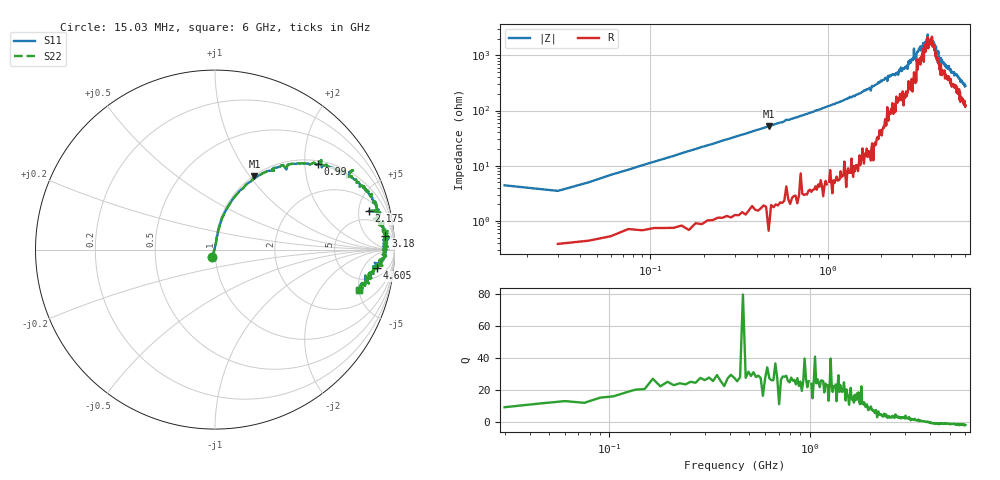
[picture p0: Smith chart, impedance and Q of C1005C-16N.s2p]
!	Network	Analyzer	HP8753E.07.74:	Oct	30	2002	Serial	No.	JP38451487
!	Hewlett-Packard
!	7	Sep	2009	8:48:05
!	Frequency	S11	S21	S12	S22
#	HZ	S	RI	R	50
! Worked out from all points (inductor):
!   400 points, 15.03 MHz to 6 GHz, reference 50 ohm
!   read as one part in series: L = 17.9 nH near 45.03 MHz
!   highest Q = 28.5 at 465 MHz (marker M1), where L = 18 nH
!   self-resonance near 3.787 GHz
!   S11 on the Smith chart (normalised r, x): 15.03 MHz: 0.97, -0.08; 990 MHz: 1.09, +2.34; 2.175 GHz: 3.30, +6.42; 3.18 GHz: 11, +18; 4.605 GHz: 9, -10; 6 GHz: 3.46, -4.99
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1.502992e7  -0.0148 -0.043  1.01 0.043  1.01 0.043  -0.0148 -0.043
3.002985e7  0.00503 0.0345  0.995 -0.0345  0.995 -0.0345  0.00503 0.0345
9.002955e7  0.0166 0.0995  0.983 -0.0995  0.983 -0.0995  0.0166 0.0995
1.95029e8  0.0531 0.205  0.947 -0.205  0.947 -0.205  0.0531 0.205
4.650277e8  0.22 0.408  0.78 -0.408  0.78 -0.408  0.22 0.408
9.90025e8  0.575 0.475  0.425 -0.475  0.425 -0.475  0.575 0.475
1.020025e9  0.591 0.471  0.409 -0.471  0.409 -0.471  0.591 0.471
2.01002e9  0.893 0.254  0.107 -0.254  0.107 -0.254  0.893 0.254
2.175019e9  0.856 0.215  0.144 -0.215  0.144 -0.215  0.856 0.215
3.015015e9  0.961 0.103  0.0388 -0.103  0.0388 -0.103  0.961 0.103
3.075015e9  0.968 0.0659  0.0318 -0.0659  0.0318 -0.0659  0.968 0.0659
3.105014e9  0.944 0.0942  0.056 -0.0942  0.056 -0.0942  0.944 0.0942
3.180014e9  0.949 0.0757  0.051 -0.0757  0.051 -0.0757  0.949 0.0757
3.585012e9  0.939 0.0337  0.0609 -0.0337  0.0609 -0.0337  0.939 0.0337
3.675012e9  0.963 0.0168  0.0367 -0.0168  0.0367 -0.0168  0.963 0.0168
3.705011e9  0.937 0.0197  0.0631 -0.0197  0.0631 -0.0197  0.937 0.0197
3.885011e9  0.956 0.000732  0.0441 -0.000732  0.0441 -0.000732  0.956 0.000732
3.91501e9  0.936 0.000366  0.0644 -0.000366  0.0644 -0.000366  0.936 0.000366
4.00501e9  0.953 -0.0354  0.0473 0.0354  0.0473 0.0354  0.953 -0.0354
4.605007e9  0.904 -0.104  0.0963 0.104  0.0963 0.104  0.904 -0.104
5.010005e9  0.878 -0.122  0.122 0.122  0.122 0.122  0.878 -0.122
6e9  0.801 -0.223  0.199 0.223  0.199 0.223  0.801 -0.223
